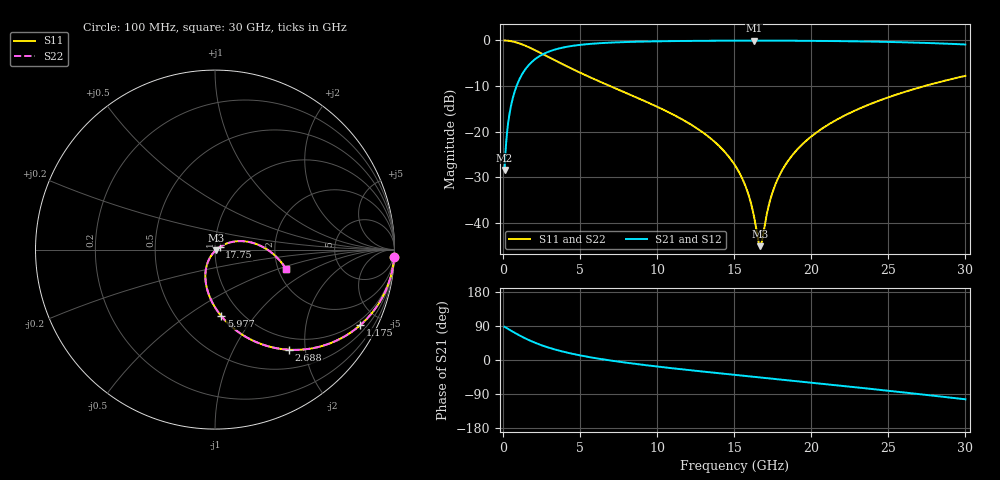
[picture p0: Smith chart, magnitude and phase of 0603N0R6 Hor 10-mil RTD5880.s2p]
# GHz S MA R 50
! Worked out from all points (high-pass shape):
!   3201 points, 100 MHz to 30 GHz, reference 50 ohm
!   highest |S21| = -0.05 dB at 16.27 GHz (marker M1); lowest = -28.4 dB at 100 MHz (marker M2)
!   |S21| within 3 dB of the highest: 2.576 GHz to end of sweep
!   lowest |S11| = -45.1 dB at 16.69 GHz (marker M3), VSWR 1.01, Z = 50.4 - j0.404 ohm
!   |S11| at or under -10 dB: 6.939 GHz to 27.35 GHz (20.41 GHz wide, 119 % of centre)
!   |S22| runs from -45.1 to 0.0 dB; largest |S21 - S12| = 0
!   S11 on the Smith chart (normalised r, x): 100 MHz: 1, -47; 1.175 GHz: 0.79, -3.95; 2.688 GHz: 0.79, -1.70; 5.977 GHz: 0.81, -0.69; 17.75 GHz: 1.05, +0.03; 30 GHz: 2.21, -0.56
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0.1  0.9992 -2.5  0.038 87.5  0.038 87.5  0.9992 -2.5
0.3335938  0.9919 -8.2  0.1257 81.8  0.1257 81.8  0.9919 -8.2
0.511125  0.9815 -12.4  0.1907 77.5  0.1907 77.5  0.9815 -12.4
1.174531  0.9125 -27.4  0.4083 62.5  0.4083 62.5  0.9125 -27.4
1.865969  0.8133 -40.8  0.5808 49.1  0.5808 49.1  0.8133 -40.8
2.688219  0.6931 -53.6  0.7193 36.3  0.7193 36.3  0.6931 -53.6
3.800125  0.5557 -66.8  0.8294 23.0  0.8294 23.0  0.5557 -66.8
5.089563  0.436 -78.2  0.8974 11.5  0.8974 11.5  0.436 -78.2
5.977219  0.3726 -84.6  0.9252 5.0  0.9252 5.0  0.3726 -84.6
10.06978  0.1852 -106.3  0.9787 -17.5  0.9787 -17.5  0.1852 -106.3
13.17191  0.09241 -118.5  0.9909 -31.4  0.9909 -31.4  0.09241 -118.5
15.05  0.04276 -122.4  0.9938 -39.3  0.9938 -39.3  0.04276 -122.4
15.76947  0.02435 -119.7  0.9942 -42.3  0.9942 -42.3  0.02435 -119.7
16.27403  0.01199 -107.3  0.9943 -44.4  0.9943 -44.4  0.01199 -107.3
16.545  0.006622 -78.9  0.9942 -45.5  0.9942 -45.5  0.006622 -78.9
16.68516  0.005563 -46.2  0.9942 -46.1  0.9942 -46.1  0.005563 -46.2
17.30184  0.01705 21.8  0.9939 -48.6  0.9939 -48.6  0.01705 21.8
17.75034  0.02843 27.7  0.9935 -50.5  0.9935 -50.5  0.02843 27.7
18.68472  0.05296 29.0  0.9923 -54.3  0.9923 -54.3  0.05296 29.0
20.03956  0.08971 25.9  0.9892 -60.0  0.9892 -60.0  0.08971 25.9
25.01978  0.2386 6.8  0.9629 -81.2  0.9629 -81.2  0.2386 6.8
30  0.4091 -15.0  0.9027 -103.7  0.9027 -103.7  0.4091 -15.0
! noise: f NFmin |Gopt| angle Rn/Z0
0.1  0.002271  0.9893  0.3715  0.04879
3.417  0.004116  0.8143  10.58  0.004591
6.743  0.006806  0.7825  19.6  0.006238
10.06  0.009281  0.7658  28.58  0.007574
13.39  0.01169  0.7562  37.46  0.008713
16.7  0.0141  0.7514  46.12  0.009713
20.03  0.01658  0.7501  54.6  0.01062
23.35  0.0192  0.7517  62.82  0.01144
26.67  0.02201  0.7556  70.82  0.01221
30  0.02507  0.7615  78.6  0.01292
